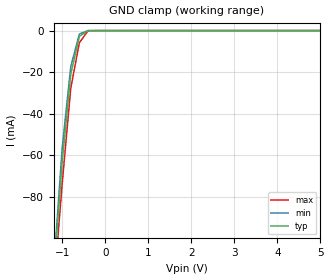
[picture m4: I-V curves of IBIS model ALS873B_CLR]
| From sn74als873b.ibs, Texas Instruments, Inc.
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|   Model ALS873B_CLR
[Model]   ALS873B_CLR
Model_type  Input
Polarity   Inverting
Vinl = 0.8
Vinh = 2.0
| variable   typ   min   max
C_comp   5.253pf   5.229pf   5.279pf
[Temperature Range]   25   0   70
[Voltage Range]   5.0   4.5   5.5
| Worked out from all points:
|   GND clamp passes 1 mA (typ) near -0.47 V on its own axis
[GND Clamp]
|   Voltage   I(typ)   I(min)   I(max)
-5V       -1.307A    -1.36A     -1.216A
-1.2V     -119.8mA   -115.6mA   -125.5mA
-1V       -63.27mA   -56.67mA   -73.91mA
-800mV    -20.91mA   -17.35mA   -27.78mA
-600mV    -2.765mA   -1.657mA   -5.861mA
-400mV    -24.85uA   -15.09uA   -133.5uA
5V        27.64pA    9.04pA     201.9pA
